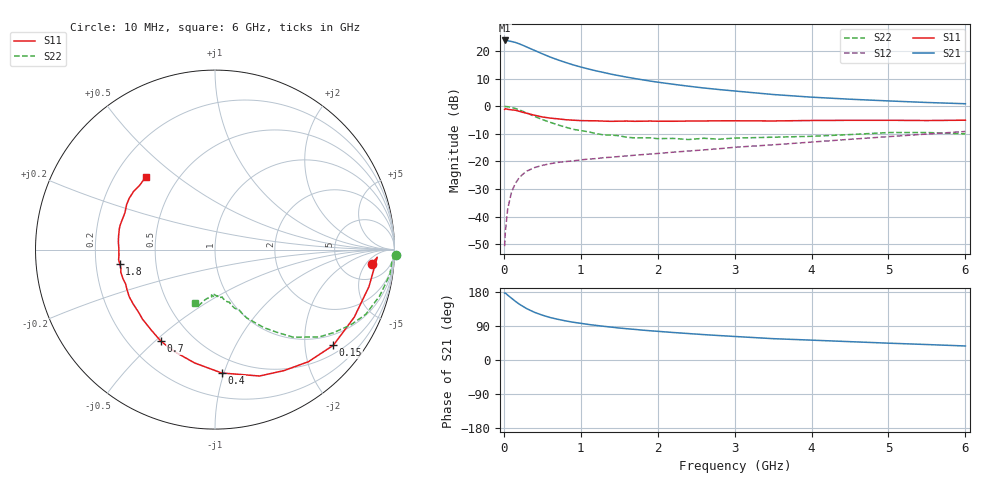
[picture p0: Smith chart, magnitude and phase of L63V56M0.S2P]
!  INFINEON TECHNOLOGIES Small Signal Semiconductors
! BFR380L3 , Si-NPN RF-Transistor in TSLP-3-1
!  Vce=3.5 V,  Ic=6 mA
! Common Emitter S-Parameters:  07. March 2005
#  GHz  S  MA  R  50
! f  S11  S21  S12  S22
! GHz  Mag  Ang  Mag  Ang  Mag  Ang  Mag  Ang
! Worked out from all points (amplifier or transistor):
!   36 points, 10 MHz to 6 GHz, reference 50 ohm
!   highest |S21| = 23.9 dB at 10 MHz (marker M1)
!   |S21| within 3 dB of that: start of sweep to 348.7 MHz
!   unconditionally stable (mu >= 1): 2.398 GHz to 4.682 GHz
!   at 250 MHz: K = 0.18, MSG = 23.3 dB, |S12| = -24.6 dB
!   at 1.4 GHz: K = 0.78, MSG = 15.1 dB, |S12| = -18.5 dB
!   at 6 GHz: K = 0.94, MSG = 5.0 dB, |S12| = -9.1 dB
!   S11 on the Smith chart (normalised r, x): 10 MHz: 10, -7; 150 MHz: 0.70, -2.66; 400 MHz: 0.38, -0.98; 700 MHz: 0.33, -0.52; 1.8 GHz: 0.30, -0.07; 6 GHz: 0.33, +0.39
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0.01  0.8769 -5.1  15.66 176.5  0.0029 78.2  1.011 -1.7
0.02  0.9049 -2.7  15.53 176.7  0.0054 93.2  0.9883 -3.3
0.05  0.8823 -13.5  15.47 171.2  0.0137 86.6  0.9843 -8.1
0.1  0.8624 -25.9  14.98 163.0  0.028 77.7  0.9532 -15.7
0.15  0.8477 -39.0  14.41 154.9  0.0398 70.8  0.9144 -23.2
0.2  0.813 -50.2  13.6 147.5  0.0508 66.1  0.8645 -29.1
0.25  0.7757 -60.4  12.74 141.3  0.0591 60.6  0.8059 -35.1
0.3  0.7466 -70.6  11.86 135.3  0.0669 57.1  0.7571 -40.0
0.4  0.6884 -86.9  10.32 125.7  0.0774 51.2  0.6547 -48.2
0.5  0.6417 -100.2  8.973 118.4  0.0848 47.8  0.5754 -53.2
0.6  0.6114 -111.7  7.849 112.2  0.0908 45.3  0.5133 -57.9
0.7  0.5928 -120.5  6.978 107.5  0.0958 44.1  0.4614 -61.5
0.9  0.5599 -136.1  5.651 99.7  0.1023 43.0  0.3825 -67.2
1.1  0.5473 -146.5  4.751 93.8  0.1103 43.5  0.3444 -71.5
1.4  0.5333 -158.8  3.815 86.7  0.1192 44.8  0.3005 -76.0
1.8  0.5366 -171.7  3.03 78.9  0.1328 47.9  0.268 -82.3
2.2  0.5355 179.5  2.513 72.6  0.1471 50.6  0.2616 -86.8
2.8  0.5454 167.9  2.013 64.5  0.1701 54.6  0.2531 -94.4
3.5  0.5422 157.8  1.637 56.3  0.2002 56.9  0.275 -99.0
4.5  0.5568 149.3  1.345 48.4  0.252 60.2  0.3069 -104.2
5.5  0.5519 139.5  1.173 40.8  0.314 60.1  0.3346 -108.8
6  0.5596 133.4  1.113 37.0  0.3491 59.0  0.3163 -111.0
